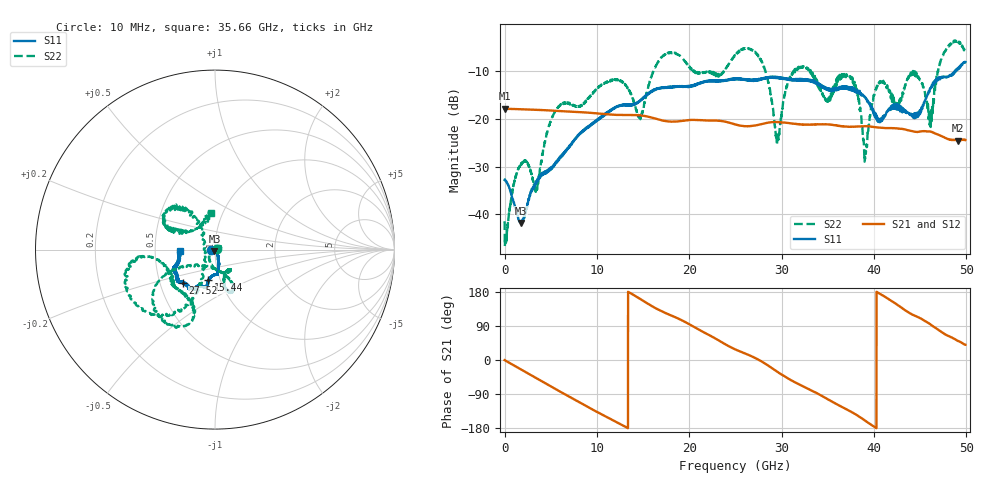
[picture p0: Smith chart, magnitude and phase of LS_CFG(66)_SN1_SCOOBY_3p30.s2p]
!Keysight Technologies,N5245B,MY58422026,A.13.80.08
!Date: Thursday, March 19, 2020 23:47:40
!Correction: S11(Full 2 Port(1,2))
!S21(Full 2 Port(1,2))
!S12(Full 2 Port(1,2))
!S22(Full 2 Port(1,2))
!S2P File: Measurements: S11, S21, S12, S22:
# Hz S DB R 50.0
!freq dBS11 angS11 dBS21 angS21 dBS12 angS12 dBS22 angS22
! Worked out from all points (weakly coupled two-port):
!   4991 points, 10 MHz to 49.91 GHz, reference 50 ohm
!   highest |S21| = -17.92 dB at 10 MHz (marker M1); lowest = -24.6 dB at 49.11 GHz (marker M2)
!   lowest |S11| = -41.8 dB at 1.77 GHz (marker M3), VSWR 1.02, Z = 49.7 - j0.737 ohm
!   |S11| at or under -10 dB: start of sweep to 48.79 GHz; 48.80968 GHz to 48.87716 GHz (67.49 MHz wide, 0.138 % of centre)
!   |S22| runs from -46.6 to -3.7 dB; largest |S21 - S12| = 0.0012
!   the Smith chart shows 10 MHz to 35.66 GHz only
!   S11 on the Smith chart (normalised r, x): 10 MHz: 0.96, -0.01; 15.44 GHz: 0.88, -0.31; 27.52 GHz: 0.65, -0.26; 35.66 GHz: 0.67, -0.01
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1e7  -32.80 -173.0  -17.92 -0.3  -17.90 -0.3  -41.43 5.9
1.77e9  -41.75 -114.7  -18.03 -24.8  -18.02 -24.8  -29.54 7.5
3.42e9  -33.21 -60.5  -18.16 -47.6  -18.15 -47.5  -35.06 136.7
5.42e9  -29.71 -61.7  -18.35 -75.3  -18.35 -75.3  -18.63 -84.2
8.33e9  -22.98 -74.1  -18.65 -114.6  -18.64 -114.5  -17.21 -62.7
1.544e10  -15.12 -102.3  -19.56 149.8  -19.55 149.9  -14.40 -152.2
1.665e10  -13.74 -102.4  -20.16 133.0  -20.16 133.1  -8.09 -147.4
2.496e10  -11.76 -124.2  -21.16 28.3  -21.15 28.5  -6.85 -171.4
2.752e10  -11.70 -133.8  -21.27 0.5  -21.27 0.8  -6.93 -125.0
2.954e10  -11.47 -141.6  -20.72 -31.0  -20.71 -30.7  -24.60 -176.3
3.103e10  -11.77 -146.6  -21.00 -53.4  -21.01 -53.1  -10.83 127.4
3.328e10  -12.11 -157.4  -21.23 -81.0  -21.23 -80.5  -10.59 156.0
3.566e10  -14.14 -178.0  -21.31 -112.3  -21.25 -111.8  -13.46 96.9
3.771e10  -14.09 171.3  -21.68 -139.2  -21.61 -139.3  -12.10 134.1
3.905e10  -15.47 169.2  -21.58 -159.9  -21.57 -160.1  -28.08 -121.3
4.03e10  -19.59 151.9  -21.82 179.8  -21.81 179.6  -13.34 -7.2
4.16e10  -17.99 103.6  -21.98 160.9  -22.00 160.9  -14.15 25.1
4.445e10  -19.26 52.2  -22.76 116.5  -22.77 116.8  -10.39 -15.8
4.614e10  -13.62 8.4  -22.69 93.6  -22.71 93.7  -21.33 -46.8
4.735e10  -11.24 8.1  -23.68 73.4  -23.69 73.6  -7.19 -83.5
4.911e10  -9.58 -14.4  -24.57 50.2  -24.59 50.3  -3.86 -44.3
4.991e10  -8.17 -15.1  -24.43 40.1  -24.46 40.2  -6.20 -28.8
